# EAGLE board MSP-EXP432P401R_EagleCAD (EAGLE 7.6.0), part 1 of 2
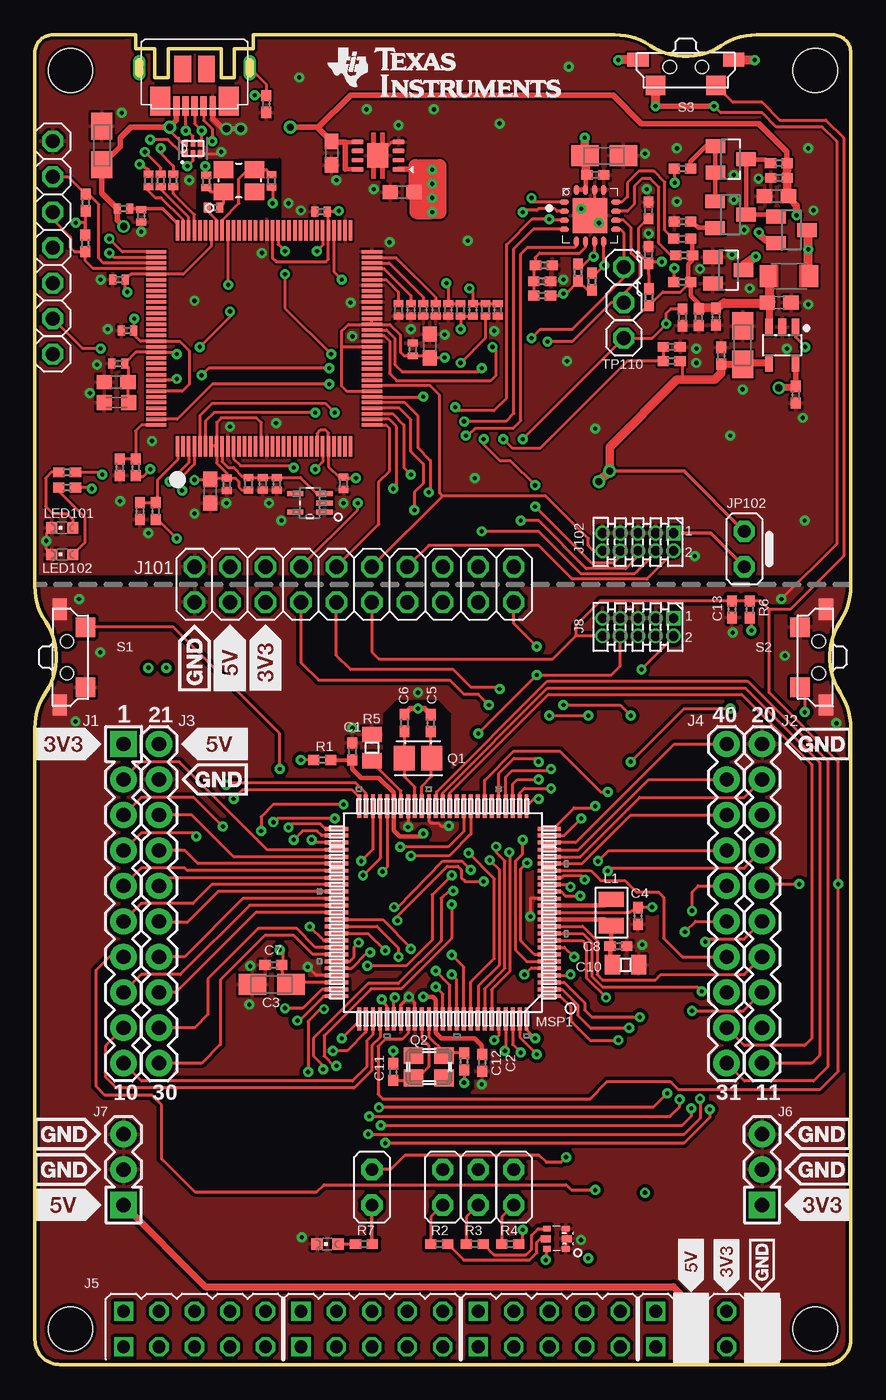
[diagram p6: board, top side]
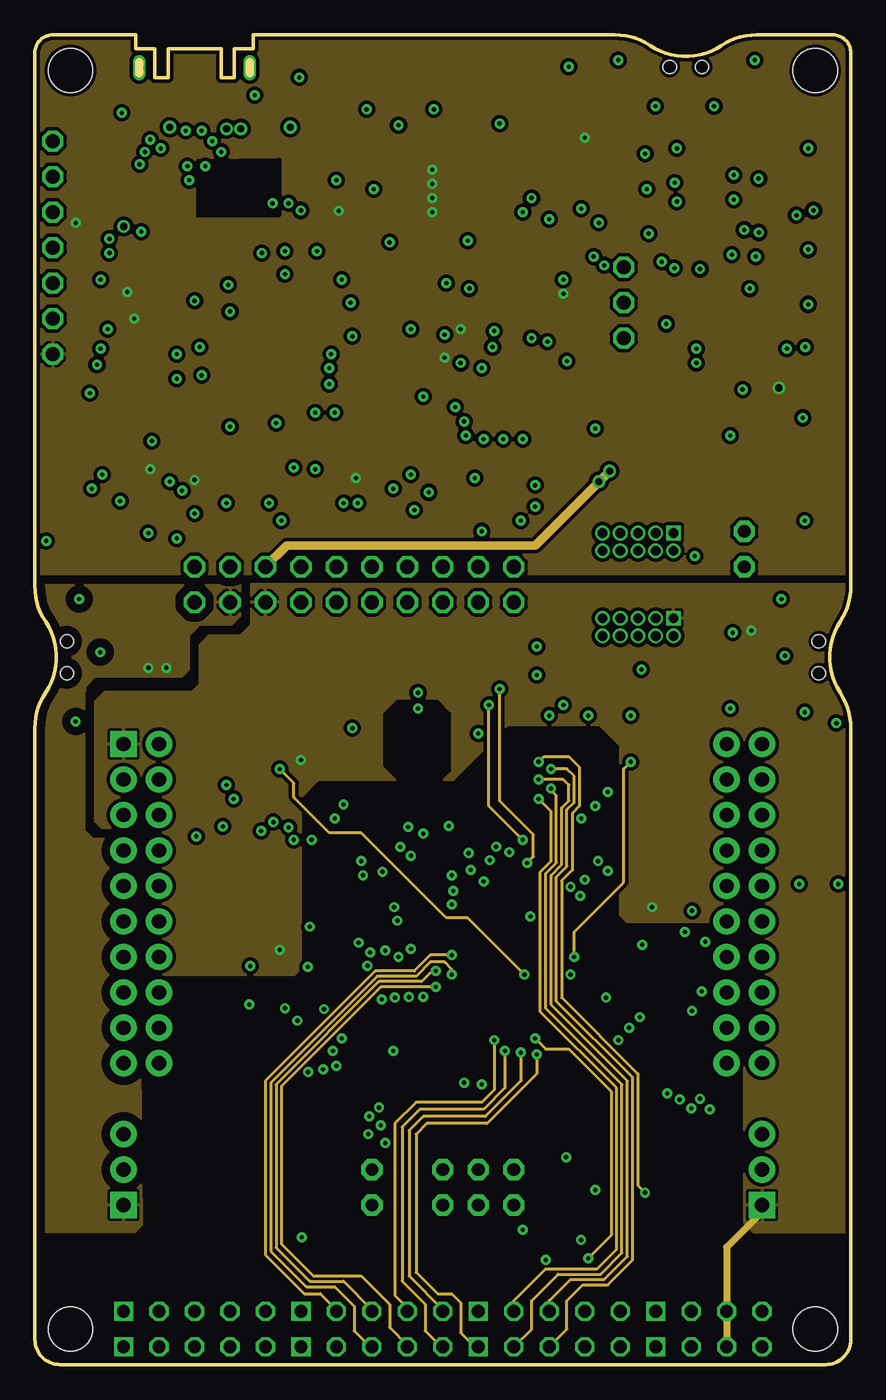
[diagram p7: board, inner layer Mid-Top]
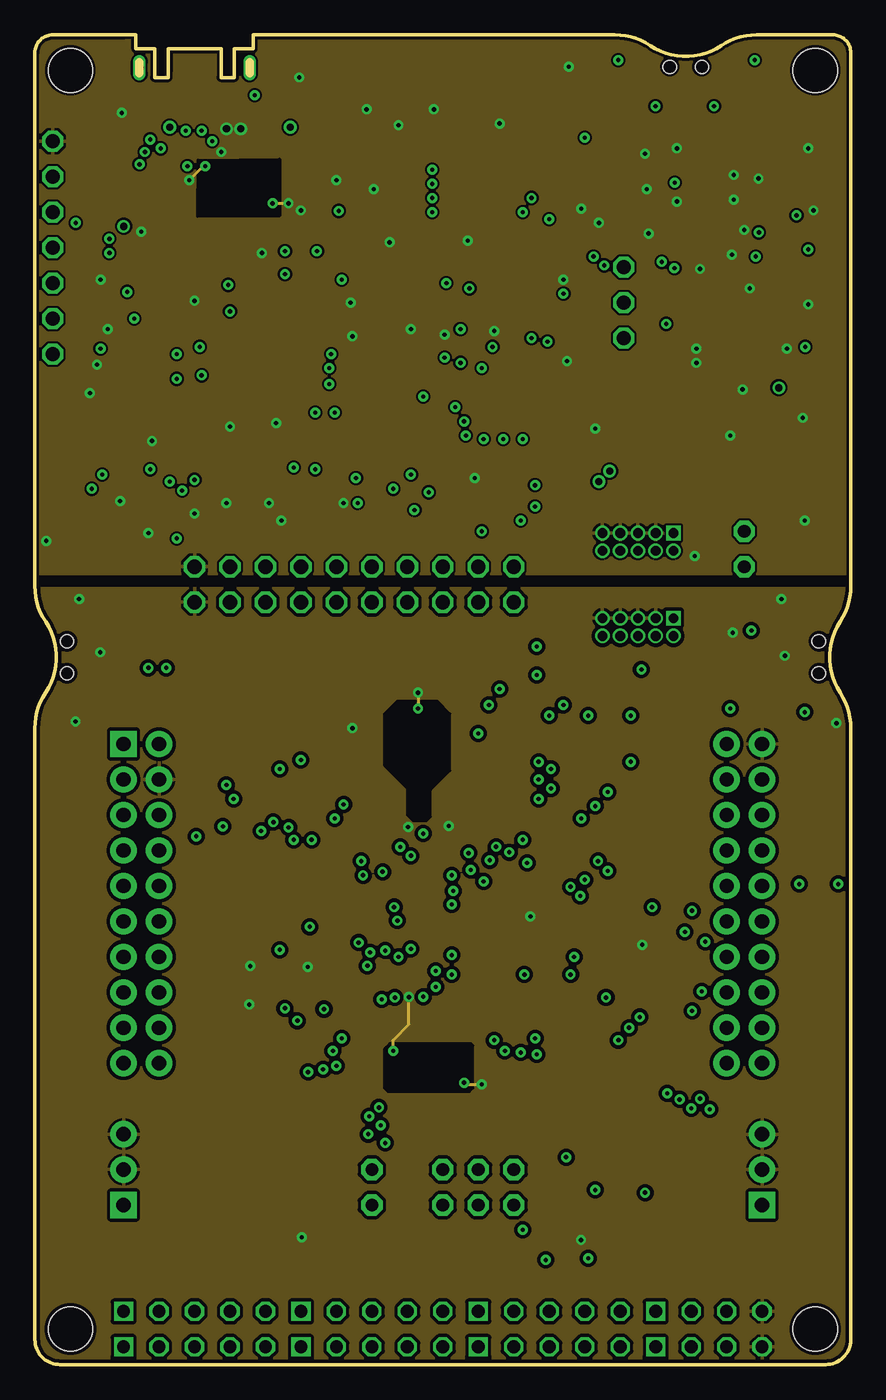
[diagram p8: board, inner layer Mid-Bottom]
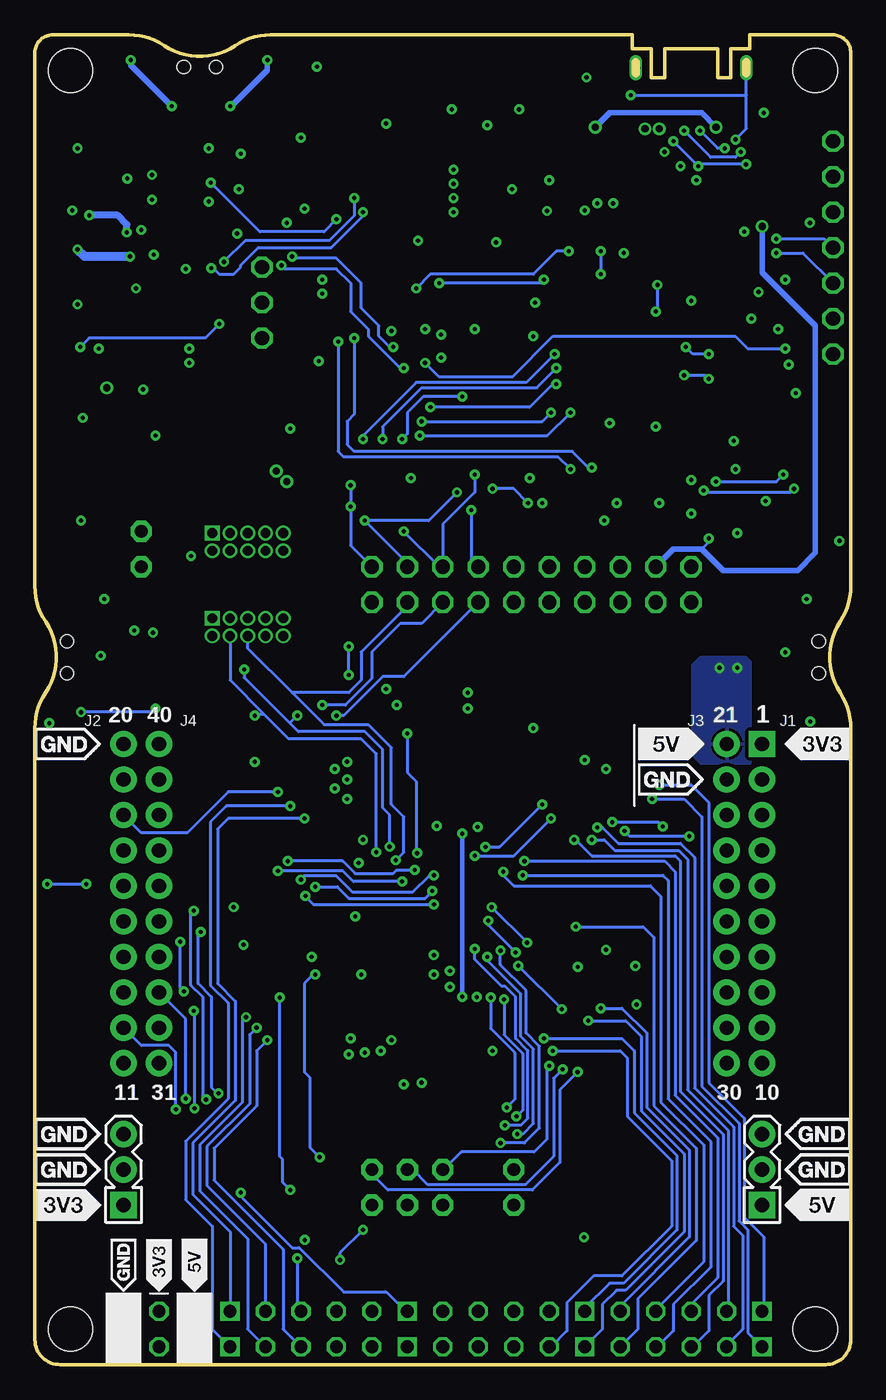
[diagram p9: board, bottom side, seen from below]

Size 58.42 x 95.25 mm. Coordinates in mm from the lower left corner, seen from the top.
Outline: 6.35,95.25 1.27,95.25 arc90 0,93.98 0,55.75 arc33 0.76,53.21 arc-67 0.76,48.13 arc33 0,45.59 0,1.8 arc90 1.8,0 56.62,0 arc90 58.42,1.78 58.42,9.27 58.42,27.3 58.42,45.59 arc33 57.66,48.13 arc-67 57.66,53.21 arc33 58.42,55.75 58.42,93.98 arc90 57.15,95.25 51.69,95.25 arc33 49.15,94.49 arc-67 44.07,94.49 arc33 41.53,95.25 16.51,95.25
Copper layers (1+2*15+16): Top 0.0178mm / dielectric 12mil / Mid-Top 0.0356mm / dielectric 27mil / Mid-Bottom 0.0356mm / dielectric 12mil / Bottom 0.0178mm
Design rules "MSP430 PCBExpress 4-layer-dietmar *": minimum track width 6mil, minimum drill 12mil, track to track 6mil, track to pad 6mil, pad to pad 6mil, via to via 8mil, smd to smd 6mil, copper to edge 8mil, drill to drill 8mil, minimum pad ring 0mil, minimum via ring 8mil, stop-mask expansion 8mil, vias tented up to drill 15mil, thermal gap 8mil
Net classes: 0 default: width 0.254 mm; 1 Ground: width 0.203 mm, drill 0.305 mm, clearance 0.152 mm to class 0, clearance 0.152 mm; 2 Power: width 0.203 mm, drill 0.305 mm, clearance 0.152 mm to class 0, clearance 0.152 mm to class 1, clearance 0.152 mm

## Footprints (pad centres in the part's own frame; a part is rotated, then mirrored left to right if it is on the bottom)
0402 = smd 0.8 x 0.7: 1 -0.6,0; 2 0.6,0
A/3216-18R = smd 1.95 x 1.5: + 1.375,0; - -1.375,0
CSMD0805 = smd 1.092 x 1.397: 1 -0.94,0; 2 0.94,0
C0402 = smd 0.5 x 0.7: 1 -0.45,0; 2 0.45,0
C0603 = smd 1.1 x 1: 1 -0.85,0; 2 0.85,0
C0603K = smd 1.05 x 1.08: 1 -0.875,0; 2 0.875,0
SOT23 = smd 1 x 1.4: 1 -0.95,-1.1; 2 0.95,-1.1; 3 0,1.1
SON8 = smd 0.85 x 0.35: 1 -1.475,0.975; 2 -1.475,0.325; 3 -1.475,-0.325; 4 -1.475,-0.975; 5 1.475,-0.975; 6 1.475,-0.325; 7 1.475,0.325; 8 1.475,0.975 | smd 1.5 x 1.75: 9 0,0
DRY6 = smd 0.559 x 0.305: 1 -0.356,0.508 | smd 0.508 x 0.305: 2 -0.381,0; 3 -0.381,-0.508; 4 0.381,-0.508; 5 0.381,0; 6 0.381,0.508
SOT23-5 = smd 0.55 x 1.2: 1 -1.204,-0.919; 2 -0.254,-0.919; 3 0.696,-0.919; 4 0.696,1.681; 5 -1.204,1.681
TQFP-128 = smd 1.45 x 0.25: P$1 0,0; P$2 0,-0.4; P$3 0,-0.8; P$4 0,-1.2; P$5 0,-1.6; P$6 0,-2; P$7 0,-2.4; P$8 0,-2.8; P$9 0,-3.2; P$10 0,-3.6; P$11 0,-4; P$12 0,-4.4; P$13 0,-4.8; P$14 0,-5.2; P$15 0,-5.6; P$16 0,-6; P$17 0,-6.4; P$18 0,-6.8; P$19 0,-7.2; P$20 0,-7.6; P$21 0,-8; P$22 0,-8.4; P$23 0,-8.8; P$24 0,-9.2; P$25 0,-9.6; P$26 0,-10; P$27 0,-10.4; P$28 0,-10.8; P$29 0,-11.2; P$30 0,-11.6; P$31 0,-12; P$32 0,-12.4; P$65 15.45,-12.4; P$66 15.45,-12; P$67 15.45,-11.6; P$68 15.45,-11.2; P$69 15.45,-10.8; P$70 15.45,-10.4; P$71 15.45,-10; P$72 15.45,-9.6; P$73 15.45,-9.2; P$74 15.45,-8.8; P$75 15.45,-8.4; P$76 15.45,-8; P$77 15.45,-7.6; P$78 15.45,-7.2; P$79 15.45,-6.8; P$80 15.45,-6.4; P$81 15.45,-6; P$82 15.45,-5.6; P$83 15.45,-5.2; P$84 15.45,-4.8; P$85 15.45,-4.4; P$86 15.45,-4; P$87 15.45,-3.6; P$88 15.45,-3.2; P$89 15.45,-2.8; P$90 15.45,-2.4; P$91 15.45,-2; P$92 15.45,-1.6; P$93 15.45,-1.2; P$94 15.45,-0.8; P$95 15.45,-0.4; P$96 15.45,0 | smd 0.25 x 1.45: P$33 1.525,-13.925; P$34 1.925,-13.925; P$35 2.325,-13.925; P$36 2.725,-13.925; P$37 3.125,-13.925; P$38 3.525,-13.925; P$39 3.925,-13.925; P$40 4.325,-13.925; P$41 4.725,-13.925; P$42 5.125,-13.925; P$43 5.525,-13.925; P$44 5.925,-13.925; P$45 6.325,-13.925; P$46 6.725,-13.925; P$47 7.125,-13.925; P$48 7.525,-13.925; P$49 7.925,-13.925; P$50 8.325,-13.925; P$51 8.725,-13.925; P$52 9.125,-13.925; P$53 9.525,-13.925; P$54 9.925,-13.925; P$55 10.325,-13.925; P$56 10.725,-13.925; P$57 11.125,-13.925; P$58 11.525,-13.925; P$59 11.925,-13.925; P$60 12.325,-13.925; P$61 12.725,-13.925; P$62 13.125,-13.925; P$63 13.525,-13.925; P$64 13.925,-13.925; P$97 13.925,1.525; P$98 13.525,1.525; P$99 13.125,1.525; P$100 12.725,1.525; P$101 12.325,1.525; P$102 11.925,1.525; P$103 11.525,1.525; P$104 11.125,1.525; P$105 10.725,1.525; P$106 10.325,1.525; P$107 9.925,1.525; P$108 9.525,1.525; P$109 9.125,1.525; P$110 8.725,1.525; P$111 8.325,1.525; P$112 7.925,1.525; P$113 7.525,1.525; P$114 7.125,1.525; P$115 6.725,1.525; P$116 6.325,1.525; P$117 5.925,1.525; P$118 5.525,1.525; P$119 5.125,1.525; P$120 4.725,1.525; P$121 4.325,1.525; P$122 3.925,1.525; P$123 3.525,1.525; P$124 3.125,1.525; P$125 2.725,1.525; P$126 2.325,1.525; P$127 1.925,1.525; P$128 1.525,1.525
DCK5 = smd 1.168 x 0.356: 1 -1.041,0.66; 2 -1.041,0; 3 -1.041,-0.66; 4 1.041,-0.66; 5 1.041,0.66
J1 = drill 1.016 pad 1.88 square: 1 0,11.43 | drill 1.016 pad 1.88: 2 0,8.89; 3 0,6.35; 4 0,3.81; 5 0,1.27; 6 0,-1.27; 7 0,-3.81; 8 0,-6.35; 9 0,-8.89; 10 0,-11.43
J2 = drill 1.016 pad 1.88: 11 0,-11.43; 12 0,-8.89; 13 0,-6.35; 14 0,-3.81; 15 0,-1.27; 16 0,1.27; 17 0,3.81; 18 0,6.35; 19 0,8.89; 20 0,11.43
J3 = drill 1.016 pad 1.88: 21 0,11.43; 22 0,8.89; 23 0,6.35; 24 0,3.81; 25 0,1.27; 26 0,-1.27; 27 0,-3.81; 28 0,-6.35; 29 0,-8.89; 30 0,-11.43
J4 = drill 1.016 pad 1.88: 31 0,-11.43; 32 0,-8.89; 33 0,-6.35; 34 0,-3.81; 35 0,-1.27; 36 0,1.27; 37 0,3.81; 38 0,6.35; 39 0,8.89; 40 0,11.43
BOTTOM_CONNECTOR = drill 0.914 square: 1 -24.13,-1.27; 2 -24.13,1.27; 11 -11.43,-1.27; 12 -11.43,1.27; 21 1.27,-1.27; 22 1.27,1.27; 31 13.97,-1.27; 32 13.97,1.27 | drill 0.914 octagon: 3 -21.59,-1.27; 4 -21.59,1.27; 5 -19.05,-1.27; 6 -19.05,1.27; 7 -16.51,-1.27; 8 -16.51,1.27; 9 -13.97,-1.27; 10 -13.97,1.27; 13 -8.89,-1.27; 14 -8.89,1.27; 15 -6.35,-1.27; 16 -6.35,1.27; 17 -3.81,-1.27; 18 -3.81,1.27; 19 -1.27,-1.27; 20 -1.27,1.27; 23 3.81,-1.27; 24 3.81,1.27; 25 6.35,-1.27; 26 6.35,1.27; 27 8.89,-1.27; 28 8.89,1.27; 29 11.43,-1.27; 30 11.43,1.27; 33 16.51,-1.27; 34 16.51,1.27; 35 19.05,-1.27; 36 19.05,1.27; 37 21.59,-1.27; 38 21.59,1.27
3PIN_PWR_3V3 = drill 1.016 pad 1.88 square: 1 0,0 | drill 1.016 pad 1.88: 2 0,2.54; 3 0,5.08
3PIN_PWR_5V = drill 1.016 pad 1.88 square: 1 0,0 | drill 1.016 pad 1.88: 2 0,2.54; 3 0,5.08
ARM-10 = drill 0.7 pad 1 square: 1 -2.54,-0.635 | drill 0.7 pad 1: 2 -2.54,0.635; 3 -1.27,-0.635; 4 -1.27,0.635; 5 0,-0.635; 6 0,0.635; 7 1.27,-0.635; 8 1.27,0.635; 9 2.54,-0.635; 10 2.54,0.635
J101_432 = drill 1.016 octagon: 1 -11.43,-1.27; 2 -11.43,1.27; 3 -8.89,-1.27; 4 -8.89,1.27; 5 -6.35,-1.27; 6 -6.35,1.27; 7 -3.81,-1.27; 8 -3.81,1.27; 9 -1.27,-1.27; 10 -1.27,1.27; 11 1.27,-1.27; 12 1.27,1.27; 13 3.81,-1.27; 14 3.81,1.27; 15 6.35,-1.27; 16 6.35,1.27; 17 8.89,-1.27; 18 8.89,1.27; 19 11.43,-1.27; 20 11.43,1.27
JP1M = drill 0.914 pad 1.524 octagon: 1 0,-1.27; 2 0,1.27
0806 = smd 1.1 x 1.8: 1 -0.94,0; 2 0.94,0
L3216C = smd 1.2 x 1.6: 1 -1.5,0; 2 1.5,0
CHIPLED_0603 = smd 0.8 x 0.8: A 0,-0.75; C 0,0.75
RGB_LED = smd 0.55 x 0.4: 1 -0.675,0.725; 3 -0.675,-0.725; 4 0.675,0.725; 6 0.675,-0.725 | smd 0.7 x 0.5: 2 -0.75,0; 5 0.75,0
PZ100 = smd 1.676 x 0.279: 1 -7.62,5.994; 2 -7.62,5.512; 3 -7.62,5.004; 4 -7.62,4.496; 5 -7.62,3.988; 6 -7.62,3.505; 7 -7.62,2.997; 8 -7.62,2.489; 9 -7.62,2.007; 10 -7.62,1.499; 11 -7.62,0.991; 12 -7.62,0.508; 13 -7.62,0; 14 -7.62,-0.508; 15 -7.62,-0.991; 16 -7.62,-1.499; 17 -7.62,-2.007; 18 -7.62,-2.489; 19 -7.62,-2.997; 20 -7.62,-3.505; 21 -7.62,-3.988; 22 -7.62,-4.496; 23 -7.62,-5.004; 24 -7.62,-5.512; 25 -7.62,-5.994; 51 7.62,-5.994; 52 7.62,-5.512; 53 7.62,-5.004; 54 7.62,-4.496; 55 7.62,-3.988; 56 7.62,-3.505; 57 7.62,-2.997; 58 7.62,-2.489; 59 7.62,-2.007; 60 7.62,-1.499; 61 7.62,-0.991; 62 7.62,-0.508; 63 7.62,0; 64 7.62,0.508; 65 7.62,0.991; 66 7.62,1.499; 67 7.62,2.007; 68 7.62,2.489; 69 7.62,2.997; 70 7.62,3.505; 71 7.62,3.988; 72 7.62,4.496; 73 7.62,5.004; 74 7.62,5.512; 75 7.62,5.994 | smd 0.279 x 1.676: 26 -5.994,-7.62; 27 -5.512,-7.62; 28 -5.004,-7.62; 29 -4.496,-7.62; 30 -3.988,-7.62; 31 -3.505,-7.62; 32 -2.997,-7.62; 33 -2.489,-7.62; 34 -2.007,-7.62; 35 -1.499,-7.62; 36 -0.991,-7.62; 37 -0.508,-7.62; 38 0,-7.62; 39 0.508,-7.62; 40 0.991,-7.62; 41 1.499,-7.62; 42 2.007,-7.62; 43 2.489,-7.62; 44 2.997,-7.62; 45 3.505,-7.62; 46 3.988,-7.62; 47 4.496,-7.62; 48 5.004,-7.62; 49 5.512,-7.62; 50 5.994,-7.62; 76 5.994,7.62; 77 5.512,7.62; 78 5.004,7.62; 79 4.496,7.62; 80 3.988,7.62; 81 3.505,7.62; 82 2.997,7.62; 83 2.489,7.62; 84 2.007,7.62; 85 1.499,7.62; 86 0.991,7.62; 87 0.508,7.62; 88 0,7.62; 89 -0.508,7.62; 90 -0.991,7.62; 91 -1.499,7.62; 92 -2.007,7.62; 93 -2.489,7.62; 94 -2.997,7.62; 95 -3.505,7.62; 96 -3.988,7.62; 97 -4.496,7.62; 98 -5.004,7.62; 99 -5.512,7.62; 100 -5.994,7.62
RSA16 = smd 0.7 x 0.35: 1 -1.85,0.975; 2 -1.85,0.325; 3 -1.85,-0.325; 4 -1.85,-0.975; 9 1.85,-0.975; 10 1.85,-0.325; 11 1.85,0.325; 12 1.85,0.975 | smd 0.35 x 0.7: 5 -0.975,-1.85; 6 -0.325,-1.85; 7 0.325,-1.85; 8 0.975,-1.85; 13 0.975,1.85; 14 0.325,1.85; 15 -0.325,1.85; 16 -0.975,1.85 | smd 2.5 x 2.5: TP 0,0
LF_XTAL = smd 1.75 x 1.5: 1 0,1; 2 0,-1
FA-238 = smd 1.4 x 1.2: 1 -1.1,-0.8; 2 1.1,-0.8; 3 1.1,0.8; 4 -1.1,0.8
NX3225GA = smd 1.4 x 1.2: 1 0,0; 2 2.2,0; 3 2.2,1.6; 4 0,1.6
0805 = smd 1.092 x 1.397: 1 -0.94,0; 2 0.94,0
R0402 = smd 0.5 x 0.7: 1 -0.45,0; 2 0.45,0
TS-1188E = smd 1.524 x 1.016: G1 -3.429,-0.508; G2 3.429,-0.508 | smd 1.397 x 1.397: S1 -2.159,1.333; S2 2.159,1.333 | hole 0.95: -1.15,0; 1.15,0
SOT23-BEC = smd 1 x 1.4: B -0.95,-1.1; C 0,1.1; E 0.95,-1.1
1X01 = drill 1.016 octagon: 1 0,0
MOUNTHOLE_125MIL = hole 3.175: 0,0
MOLEX_105164-0001 = smd 0.45 x 1.4: D+ 0,-4.1; D- -0.65,-4.1; GND 1.3,-4.1; ID 0.65,-4.1; VBUS -1.3,-4.1 | smd 1.45 x 2.1: SHIELD1 -2.45,-3.75; SHIELD4 2.45,-3.75 | smd 1.2 x 1.9: SHIELD2 -0.85,-1.45; SHIELD3 0.85,-1.45 | drill 0.6 long: SHIELD_TH1 -3.95,-1.35; SHIELD_TH2 3.95,-1.35

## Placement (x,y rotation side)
C1  100n  [0402]  22.73,43.92 90 top
C2  100n  [0402]  32.03,21.62 270 top
C3  10u  [A/3216-18R]  16.95,27.24 0 top
C4  100n  [0402]  43.18,32.13 270 top
C5  22p  [0402]  28.35,45.95 90 top
C6  22p  [0402]  26.47,45.97 90 top
C7  100n  [0402]  17.08,28.64 180 top
C8  100n  [0402]  41.78,29.97 0 top
C10  4u7  [CSMD0805]  42.29,28.64 0 top
C11  22p  [0402]  25.65,20.96 90 top
C12  22p  [0402]  30.73,21.72 270 top
C13  1n  [0402]  49.91,54.1 270 top
C101  12pF  [C0402]  12.27,84.76 90 top
C102  12pF  [C0402]  16.94,84.79 270 top
C103  0.1uF  [C0402]  29.59,75.56 270 top
C104  10n  [C0402]  13.74,63.04 270 top
C105  2u2  [C0603]  26.29,83.98 180 top
C106  4.7u  [A/3216-18R]  40.77,86.58 180 top
C107  1u  [C0603]  12.55,62.56 270 top
C108  DNP  [C0402]  33.15,75.56 270 top
C110  10n  [C0402]  17.32,63.09 270 top
C111  100n  [C0402]  16.31,63.09 270 top
C112  10n  [C0402]  22.1,63.12 270 top
C113  100n  [C0402]  27.05,72.71 90 top
C114  10n  [C0402]  6.62,74.07 180 top
C115  33p  [0402]  43.94,82.68 270 top
C116  33p  [0402]  36.45,78.74 180 top
C117  4.7u  [C0603]  53.1,83.7 180 top
C118  100n  [0402]  53.28,85 180 top
C119  4.7u  [C0603]  53.29,76.06 0 top
C120  100n  [0402]  47.53,75.03 270 top
C121  100n  [C0402]  20.47,82.58 180 top
C123  10n  [C0402]  6.03,77.72 180 top
C124  100n  [0402]  40.13,85.22 0 top
C126  220n  [0402]  54.48,69.47 270 top
C127  220n  [0402]  48.77,75.06 270 top
C128  47u  [A/3216-18R]  50.67,73.03 270 top
C129  100n  [0402]  49.15,72.26 90 top
C130  1u  [C0603]  28.26,72.96 270 top
C131  0.1uF  [C0402]  5.97,71.7 180 top
C132  1u  [C0603]  5.82,70.38 0 top
C133  2.2uF  [C0603K]  5.84,68.91 180 top
C140  4.7u  [A/3216-18R]  4.8,87.33 270 top
C141  1u  [C0603]  21.24,86.78 270 top
C150  0.1uF  [C0402]  7.62,82.3 270 top
D101  BAS40-05  [SOT23]  49.82,86.34 270 top
D102  BAS40-05  [SOT23]  49.65,78.39 270 top
IC101  TPS73533DRB  [SON8]  24.56,86.6 180 top
IC102  TPD4E004_DRY_6  [DRY6]  11.32,87.12 90 top
IC103  TPS2102DBV  [SOT23-5]  53.26,73.41 180 top
IC106  TM4C129ENCPDT  [TQFP-128]  10.21,65.79 90 top
IC107  LM4040B25_DCK_5  [DCK5]  19.68,61.72 180 top
J1  [J1]  6.35,33.02 0 top
J2  [J2]  52.07,33.02 0 top
J3  [J3]  8.89,33.02 0 top
J4  [J4]  49.53,33.02 0 top
J5  EDGE_CON  [BOTTOM_CONNECTOR]  30.48,2.54 0 top
J6  HEADER 1X03  [3PIN_PWR_3V3]  52.07,11.43 0 top
J7  BP_HEADERS_PWR_5V  [3PIN_PWR_5V]  6.35,11.43 0 top
J8  [ARM-10]  43.18,52.83 180 top
J101  J101_432  [J101_432]  22.86,55.88 0 top
J102  [ARM-10]  43.18,58.93 180 top
JP8  LED1  [JP1M]  24.13,12.7 180 top
JP9  LED2_RED  [JP1M]  29.21,12.7 180 top
JP10  LED2_GREEN  [JP1M]  31.75,12.7 180 top
JP11  LED2_BLUE  [JP1M]  34.29,12.7 180 top
JP102  [JP1M]  50.8,58.42 180 top
L1  4.7uH  [0806]  41.27,32.38 90 top
L101  2u2  [L3216C]  53.99,77.97 180 top
LED1  [CHIPLED_0603]  20.96,8.64 90 top
LED2  EVERLIGHT_19-337  [RGB_LED]  37.34,9.02 180 top
LED101  [CHIPLED_0603]  1.97,59.94 90 top
LED102  [CHIPLED_0603]  1.97,58.03 90 top
MSP1  MSP432  [PZ100]  29.21,32.38 180 top
MSP101  MSP430G2452IRSA16R  [RSA16]  39.75,82.3 0 top
Q1  [LF_XTAL]  27.43,43.43 90 top
Q2  [FA-238]  28.19,21.34 180 top
Q101  NX3225GA_OSC  [NX3225GA]  13.51,84 0 top
R1  0R  [0402]  20.57,43.31 0 top
R2  110R  [0402]  28.96,8.64 0 top
R3  16R  [0402]  31.5,8.64 0 top
R4  24R  [0402]  34.04,8.64 0 top
R5  91kOhm, 0.1%, 25ppm/C  [0805]  24.13,44.2 90 top
R6  47k  [0402]  51.18,54.1 270 top
R7  470  [0402]  23.56,8.64 180 top
R101  DNP  [0402]  45.59,72.9 180 top
R102  100  [R0402]  32.26,75.56 90 top
R103  10k  [R0402]  31.37,75.56 90 top
R104  51  [R0402]  30.48,75.56 90 top
R105  1k 1%  [R0402]  15.29,63.09 270 top
R106  2R  [R0402]  12.78,82.88 180 top
R107  47k  [0402]  46.37,75.01 270 top
R108  1k  [R0402]  28.7,75.56 90 top
R109  1k  [R0402]  27.81,75.56 90 top
R110  1k  [R0402]  26.92,75.56 90 top
R111  470  [0402]  2.31,63.92 180 top
R112  220k  [0402]  43.97,76.45 90 top
R113  220k  [0402]  43.95,79.48 90 top
R114  220k  [0402]  36.32,76.58 180 top
R115  220k  [0402]  36.32,77.6 0 top
R116  4k7  [0402]  39.89,77.58 90 top
R117  4k7  [0402]  38.9,78.22 90 top
R118  820  [0402]  46.37,85.66 180 top
R119  0  [0402]  46.37,81.88 180 top
R120  470  [0402]  53.28,86.07 180 top
R123  33  [0402]  16.56,90.29 270 top
R124  470  [0402]  2.31,62.83 180 top
R125  10k  [0402]  3.63,83.24 270 top
R126  2k2  [0402]  46.35,80.64 180 top
R127  3k3  [0402]  46.35,77.55 180 top
R128  6k8  [0402]  46.48,79.45 180 top
R129  10k  [0402]  3.61,80.31 90 top
R131  0  [R0402]  8.13,84.84 270 top
R132  330k  [0402]  8.66,61.14 90 top
R133  220k  [0402]  7.52,61.14 90 top
R134  DNP  [0402]  45.59,71.88 180 top
R135  220k  [0402]  7.21,64.27 90 top
R136  220k  [0402]  6.07,64.27 90 top
R137  0  [R0402]  9.02,84.84 270 top
R138  0  [R0402]  9.91,84.84 270 top
R139  dnp  [R0402]  26.04,75.56 90 top
R140  51  [R0402]  6.35,82.8 0 top
S1  [TS-1188E]  2.29,50.67 270 top
S2  [TS-1188E]  56.13,50.67 90 top
S3  [TS-1188E]  46.61,92.96 180 top
T101  DMG1013UW  [SOT23]  54.17,81.27 270 top
T102  BC850CW-115  [SOT23-BEC]  49.81,82.37 270 top
TP101  TEST_PIN2  [1X01]  1.27,87.63 270 top
TP102  TEST_PIN2  [1X01]  1.27,85.09 270 top
TP103  TEST_PIN2  [1X01]  1.27,82.55 270 top
TP104  TEST_PIN2  [1X01]  1.27,80.01 270 top
TP105  TEST_PIN2  [1X01]  1.27,77.47 270 top
TP106  TEST_PIN2  [1X01]  1.27,74.93 270 top
TP107  TEST_PIN2  [1X01]  1.27,72.39 0 top
TP108  TEST_PIN2  [1X01]  42.16,78.61 0 top
TP109  TEST_PIN2  [1X01]  42.16,76.07 0 top
TP110  TEST_PIN2  [1X01]  42.16,73.53 0 top
U$1  MOUNTHOLE_125MIL  [MOUNTHOLE_125MIL]  2.54,2.54 0 top
U$2  MOUNTHOLE_125MIL  [MOUNTHOLE_125MIL]  55.88,2.54 0 top
U$3  MOUNTHOLE_125MIL  [MOUNTHOLE_125MIL]  2.54,92.71 0 top
U$4  [LOGO16_TPLACE]  20.89,90.63 0 top
U$5  MOUNTHOLE_125MIL  [MOUNTHOLE_125MIL]  55.88,92.71 0 top
U$7  MIKE_TM  [MIKE_TM]  29.21,31.11 0 top
U$8  P401R_REARSILK_REV2_1  [P401R_REARSILK_REV2_1]  0,55.88 0 top
U$9  REAR_TILOGO  [REAR_TILOGO]  16.64,30.78 0 top
U$10  COMPLIANCE_SUITESYMBOLONLY  [EVM_COMPLIANCESUITE_SYMBOLONLY]  18.8,5.38 0 top
U$11  COMPLIANCE_FCC_TEXTREAR  [COMPLIANCE_FCC_TEXT]  19.05,4.83 0 top
U$12  LOGO-ROCKET  [LOGO-ROCKET]  10.03,12.95 0 top
U$13  P401R_SILKLABEL  [SILKLABELUPDATED]  45.72,0 0 top
USB101  [MOLEX_105164-0001]  11.43,94.25 0 top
